DATA_BLOCK DB 24
AUTHOR : Esposito
FAMILY : EGAL_srl
NAME : DB_KEY_O
VERSION : 0.1


  STRUCT
   key_0_0 : BOOL ;
   key_0_1 : BOOL ;
   key_0_2 : BOOL ;
   key_0_3 : BOOL ;
   key_0_4 : BOOL ;
   key_0_5 : BOOL ;
   key_0_6 : BOOL ;
   key_0_7 : BOOL ;
   key_1_0 : BOOL ;
   key_1_1 : BOOL ;
   key_1_2 : BOOL ;
   key_1_3 : BOOL ;
   key_1_4 : BOOL ;
   key_1_5 : BOOL ;
   key_1_6 : BOOL ;
   key_1_7 : BOOL ;
   key_2_0 : BOOL ;
   key_2_1 : BOOL ;
   key_2_2 : BOOL ;
   key_2_3 : BOOL ;
   key_2_4 : BOOL ;
   key_2_5 : BOOL ;
   key_2_6 : BOOL ;
   key_2_7 : BOOL ;
   key_3_0 : BOOL ;
   key_3_1 : BOOL ;
   key_3_2 : BOOL ;
   key_3_3 : BOOL ;
   key_3_4 : BOOL ;
   key_3_5 : BOOL ;
   key_3_6 : BOOL ;
   key_3_7 : BOOL ;
   key_4_0 : BOOL ;
   key_4_1 : BOOL ;
   key_4_2 : BOOL ;
   key_4_3 : BOOL ;
   key_4_4 : BOOL ;
   key_4_5 : BOOL ;
   key_4_6 : BOOL ;
   key_4_7 : BOOL ;
   key_5_0 : BOOL ;
   key_5_1 : BOOL ;
   key_5_2 : BOOL ;
   key_5_3 : BOOL ;
   key_5_4 : BOOL ;
   key_5_5 : BOOL ;
   key_5_6 : BOOL ;
   key_5_7 : BOOL ;
   key_6_0 : BOOL ;
   key_6_1 : BOOL ;
   key_6_2 : BOOL ;
   key_6_3 : BOOL ;
   key_6_4 : BOOL ;
   key_6_5 : BOOL ;
   key_6_6 : BOOL ;
   key_6_7 : BOOL ;
   key_7_0 : BOOL ;
   key_7_1 : BOOL ;
   key_7_2 : BOOL ;
   key_7_3 : BOOL ;
   key_7_4 : BOOL ;
   key_7_5 : BOOL ;
   key_7_6 : BOOL ;
   key_7_7 : BOOL ;
   key_8_0 : BOOL ;
   key_8_1 : BOOL ;
   key_8_2 : BOOL ;
   key_8_3 : BOOL ;
   key_8_4 : BOOL ;
   key_8_5 : BOOL ;
   key_8_6 : BOOL ;
   key_8_7 : BOOL ;
   key_9_0 : BOOL ;
   key_9_1 : BOOL ;
   key_9_2 : BOOL ;
   key_9_3 : BOOL ;
   key_9_4 : BOOL ;
   key_9_5 : BOOL ;
   key_9_6 : BOOL ;
   key_9_7 : BOOL ;
   key_10_0 : BOOL ;
   key_10_1 : BOOL ;
   key_10_2 : BOOL ;
   key_10_3 : BOOL ;
   key_10_4 : BOOL ;
   key_10_5 : BOOL ;
   key_10_6 : BOOL ;
   key_10_7 : BOOL ;
   key_11_0 : BOOL ;
   key_11_1 : BOOL ;
   key_11_2 : BOOL ;
   key_11_3 : BOOL ;
   key_11_4 : BOOL ;
   key_11_5 : BOOL ;
   key_11_6 : BOOL ;
   key_11_7 : BOOL ;
   key_12_0 : BOOL ;
   key_12_1 : BOOL ;
   key_12_2 : BOOL ;
   key_12_3 : BOOL ;
   key_12_4 : BOOL ;
   key_12_5 : BOOL ;
   key_12_6 : BOOL ;
   key_12_7 : BOOL ;
   key_13_0 : BOOL ;
   key_13_1 : BOOL ;
   key_13_2 : BOOL ;
   key_13_3 : BOOL ;
   key_13_4 : BOOL ;
   key_13_5 : BOOL ;
   key_13_6 : BOOL ;
   key_13_7 : BOOL ;
   key_14_0 : BOOL ;
   key_14_1 : BOOL ;
   key_14_2 : BOOL ;
   key_14_3 : BOOL ;
   key_14_4 : BOOL ;
   key_14_5 : BOOL ;
   key_14_6 : BOOL ;
   key_14_7 : BOOL ;
   key_15_0 : BOOL ;
   key_15_1 : BOOL ;
   key_15_2 : BOOL ;
   key_15_3 : BOOL ;
   key_15_4 : BOOL ;
   key_15_5 : BOOL ;
   key_15_6 : BOOL ;
   key_15_7 : BOOL ;
   key_16_0 : BOOL ;
   key_16_01 : BOOL ;
   key_16_02 : BOOL ;
   key_16_03 : BOOL ;
   key_16_04 : BOOL ;
   key_16_05 : BOOL ;
   key_16_06 : BOOL ;
   key_16_07 : BOOL ;
   key_17_0 : BOOL ;
   key_17_01 : BOOL ;
   key_17_02 : BOOL ;
   key_17_03 : BOOL ;
   key_17_04 : BOOL ;
   key_17_05 : BOOL ;
   key_17_06 : BOOL ;
   key_17_07 : BOOL ;
   key_18_0 : BOOL ;
   key_18_1 : BOOL ;
   key_18_2 : BOOL ;
   key_18_3 : BOOL ;
   key_18_4 : BOOL ;
   key_18_5 : BOOL ;
   key_18_6 : BOOL ;
   key_18_7 : BOOL ;
  END_STRUCT ;
BEGIN
   key_0_0 := FALSE;
   key_0_1 := FALSE;
   key_0_2 := FALSE;
   key_0_3 := FALSE;
   key_0_4 := FALSE;
   key_0_5 := FALSE;
   key_0_6 := FALSE;
   key_0_7 := FALSE;
   key_1_0 := FALSE;
   key_1_1 := FALSE;
   key_1_2 := FALSE;
   key_1_3 := FALSE;
   key_1_4 := FALSE;
   key_1_5 := FALSE;
   key_1_6 := FALSE;
   key_1_7 := FALSE;
   key_2_0 := FALSE;
   key_2_1 := FALSE;
   key_2_2 := FALSE;
   key_2_3 := FALSE;
   key_2_4 := FALSE;
   key_2_5 := FALSE;
   key_2_6 := FALSE;
   key_2_7 := FALSE;
   key_3_0 := FALSE;
   key_3_1 := FALSE;
   key_3_2 := FALSE;
   key_3_3 := FALSE;
   key_3_4 := FALSE;
   key_3_5 := FALSE;
   key_3_6 := FALSE;
   key_3_7 := FALSE;
   key_4_0 := FALSE;
   key_4_1 := FALSE;
   key_4_2 := FALSE;
   key_4_3 := FALSE;
   key_4_4 := FALSE;
   key_4_5 := FALSE;
   key_4_6 := FALSE;
   key_4_7 := FALSE;
   key_5_0 := FALSE;
   key_5_1 := FALSE;
   key_5_2 := FALSE;
   key_5_3 := FALSE;
   key_5_4 := FALSE;
   key_5_5 := FALSE;
   key_5_6 := FALSE;
   key_5_7 := FALSE;
   key_6_0 := FALSE;
   key_6_1 := FALSE;
   key_6_2 := FALSE;
   key_6_3 := FALSE;
   key_6_4 := FALSE;
   key_6_5 := FALSE;
   key_6_6 := FALSE;
   key_6_7 := FALSE;
   key_7_0 := FALSE;
   key_7_1 := FALSE;
   key_7_2 := FALSE;
   key_7_3 := FALSE;
   key_7_4 := FALSE;
   key_7_5 := FALSE;
   key_7_6 := FALSE;
   key_7_7 := FALSE;
   key_8_0 := FALSE;
   key_8_1 := FALSE;
   key_8_2 := FALSE;
   key_8_3 := FALSE;
   key_8_4 := FALSE;
   key_8_5 := FALSE;
   key_8_6 := FALSE;
   key_8_7 := FALSE;
   key_9_0 := FALSE;
   key_9_1 := FALSE;
   key_9_2 := FALSE;
   key_9_3 := FALSE;
   key_9_4 := FALSE;
   key_9_5 := FALSE;
   key_9_6 := FALSE;
   key_9_7 := FALSE;
   key_10_0 := FALSE;
   key_10_1 := FALSE;
   key_10_2 := FALSE;
   key_10_3 := FALSE;
   key_10_4 := FALSE;
   key_10_5 := FALSE;
   key_10_6 := FALSE;
   key_10_7 := FALSE;
   key_11_0 := FALSE;
   key_11_1 := FALSE;
   key_11_2 := FALSE;
   key_11_3 := FALSE;
   key_11_4 := FALSE;
   key_11_5 := FALSE;
   key_11_6 := FALSE;
   key_11_7 := FALSE;
   key_12_0 := FALSE;
   key_12_1 := FALSE;
   key_12_2 := FALSE;
   key_12_3 := FALSE;
   key_12_4 := FALSE;
   key_12_5 := FALSE;
   key_12_6 := FALSE;
   key_12_7 := FALSE;
   key_13_0 := FALSE;
   key_13_1 := FALSE;
   key_13_2 := FALSE;
   key_13_3 := FALSE;
   key_13_4 := FALSE;
   key_13_5 := FALSE;
   key_13_6 := FALSE;
   key_13_7 := FALSE;
   key_14_0 := FALSE;
   key_14_1 := FALSE;
   key_14_2 := FALSE;
   key_14_3 := FALSE;
   key_14_4 := FALSE;
   key_14_5 := FALSE;
   key_14_6 := FALSE;
   key_14_7 := FALSE;
   key_15_0 := FALSE;
   key_15_1 := FALSE;
   key_15_2 := FALSE;
   key_15_3 := FALSE;
   key_15_4 := FALSE;
   key_15_5 := FALSE;
   key_15_6 := FALSE;
   key_15_7 := FALSE;
   key_16_0 := FALSE;
   key_16_01 := FALSE;
   key_16_02 := FALSE;
   key_16_03 := FALSE;
   key_16_04 := FALSE;
   key_16_05 := FALSE;
   key_16_06 := FALSE;
   key_16_07 := FALSE;
   key_17_0 := FALSE;
   key_17_01 := FALSE;
   key_17_02 := FALSE;
   key_17_03 := FALSE;
   key_17_04 := FALSE;
   key_17_05 := FALSE;
   key_17_06 := FALSE;
   key_17_07 := FALSE;
   key_18_0 := FALSE;
   key_18_1 := FALSE;
   key_18_2 := FALSE;
   key_18_3 := FALSE;
   key_18_4 := FALSE;
   key_18_5 := FALSE;
   key_18_6 := FALSE;
   key_18_7 := FALSE;
END_DATA_BLOCK

